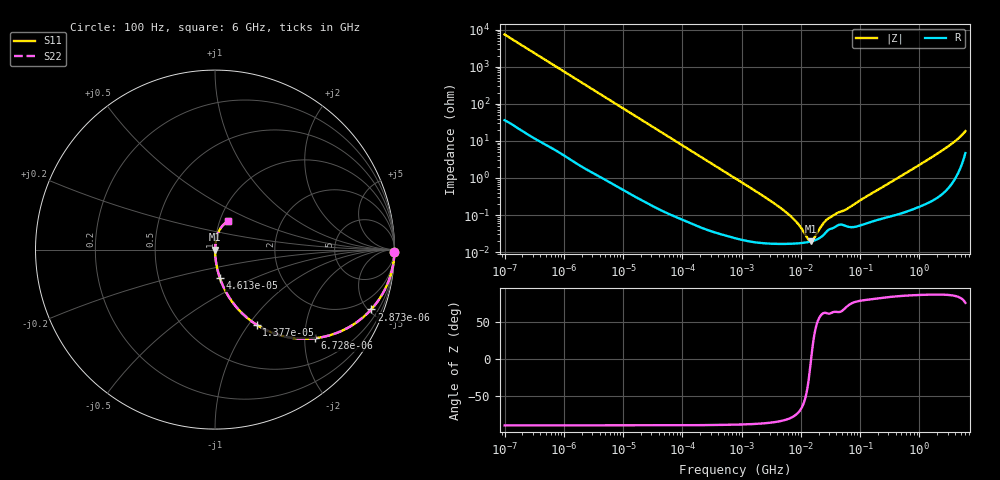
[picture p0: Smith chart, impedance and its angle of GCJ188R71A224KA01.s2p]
!Murata Part Number: GCJ188R71A224KA01
!These Parameters are Measured in Series Mode Connection
!Data Generated on Mar 13, 2026
!  o--ll--o
!Port1  Port2
!  o------o
!Operation Temp=25[degC], DC Bias Voltage=0[V]
!Freq. Start=100[Hz] Stop=6[GHz] 401[Steps]
# Hz S RI R 50
!Freq.(Hz) S11(Real) S11(Imag) S21(Real) S21(Imag) S12(Real) S12(Imag) S22(Real) S22(Imag)
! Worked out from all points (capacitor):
!   401 points, 100 Hz to 6 GHz, reference 50 ohm
!   read as one part in series: C = 214 nF near 109 Hz
!   lowest |Z| = 19.4 mohm at 14.88 MHz (marker M1)
!   series resonance near 14.95 MHz, so ESL is about 530 pH
!   S11 on the Smith chart (normalised r, x): 100 Hz: open; 2.873 kHz: 1.03, -5.21; 6.728 kHz: 1.01, -2.23; 13.77 kHz: 1.01, -1.09; 46.13 kHz: 1.00, -0.33; 6 GHz: 1.09, +0.35
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100  0.9998 -0.0135  0.000248 0.0135  0.000248 0.0135  0.9998 -0.0135
600  0.9931 -0.0799  0.00685 0.0799  0.00685 0.0799  0.9931 -0.0799
2008  0.9317 -0.2497  0.0683 0.2497  0.0683 0.2497  0.9317 -0.2497
2873  0.8704 -0.3331  0.1296 0.3331  0.1296 0.3331  0.8704 -0.3331
6728  0.5548 -0.494  0.4452 0.494  0.4452 0.494  0.5548 -0.494
13772  0.2319 -0.4188  0.7681 0.4188  0.7681 0.4188  0.2319 -0.4188
22537  0.1026 -0.3  0.8974 0.3  0.8974 0.3  0.1026 -0.3
40335  0.0353 -0.1808  0.9647 0.1808  0.9647 0.1808  0.0353 -0.1808
46134  0.0274 -0.1594  0.9726 0.1594  0.9726 0.1594  0.0274 -0.1594
141303  0.00348 -0.0537  0.9965 0.0537  0.9965 0.0537  0.00348 -0.0537
774597  0.000336 -0.0099  0.9997 0.0099  0.9997 0.0099  0.000336 -0.0099
5809218  0.000168 -0.00113  0.9998 0.00113  0.9998 0.00113  0.000168 -0.00113
8692127  0.000172 -0.000591  0.9998 0.000591  0.9998 0.000591  0.000172 -0.000591
1.300572e7  0.000185 -0.000146  0.9998 0.000146  0.9998 0.000146  0.000185 -0.000146
1.487547e7  0.000194 -5.2e-06  0.9998 5.2e-06  0.9998 5.2e-06  0.000194 -5.2e-06
1.555665e7  0.000198 4.18e-05  0.9998 -4.18e-05  0.9998 -4.18e-05  0.000198 4.18e-05
2.327686e7  0.000274 0.000486  0.9997 -0.000486  0.9997 -0.000486  0.000274 0.000486
2.911731e7  0.000396 0.000703  0.9996 -0.000703  0.9996 -0.000703  0.000396 0.000703
5.960426e7  0.000496 0.00136  0.9995 -0.00136  0.9995 -0.00136  0.000496 0.00136
3.124326e8  0.000947 0.00723  0.9991 -0.00723  0.9991 -0.00723  0.000947 0.00723
2.34314e9  0.00622 0.0523  0.9938 -0.0523  0.9938 -0.0523  0.00622 0.0523
6e9  0.0716 0.1572  0.9284 -0.1572  0.9284 -0.1572  0.0716 0.1572
